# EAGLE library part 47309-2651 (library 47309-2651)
1 Micro SD Detect switch 2.65mm height Source: Datasheet
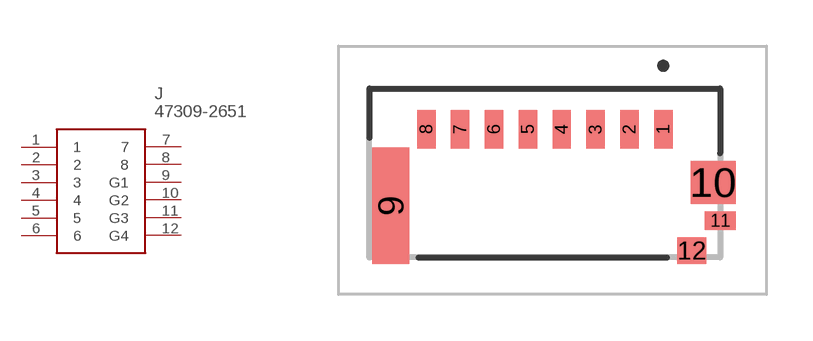
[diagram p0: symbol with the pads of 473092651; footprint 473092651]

Designator prefix J

## 47309-2651 (Description: 1 Micro SD Detect switch 2.65mm height; Height: 2.65mm; Manufacturer_Name: Molex; Manufacturer_Part_Number: 47309-2651; Mouser_Part_Number: 538-47309-2651; Mouser_Price-Stock: https://www.mouser.co.uk/ProductDetail/Molex/47309-2651?qs=%252Bi0aAQIdfgCnu2Vhp4wRvw%3D%3D)  [473092651]
1  1
2  2
3  3
4  4
5  5
6  6
7  7
8  8
9  G1
10  G2
11  G3
12  G4

## Footprint 473092651 (pad centres in mm)
47309-2651
smd 0.6 x 1.25: 1 3.6,1.333; 2 2.5,1.333; 3 1.4,1.333; 4 0.3,1.333; 5 -0.8,1.333; 6 -1.9,1.333; 7 -3,1.333; 8 -4.1,1.333
smd 1.2 x 3.79: 9 -5.25,-1.147
smd 1.45 x 1.4: 10 5.225,-0.392
smd 1 x 0.6: 11 5.45,-1.642
smd 0.95 x 0.85: 12 4.525,-2.617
